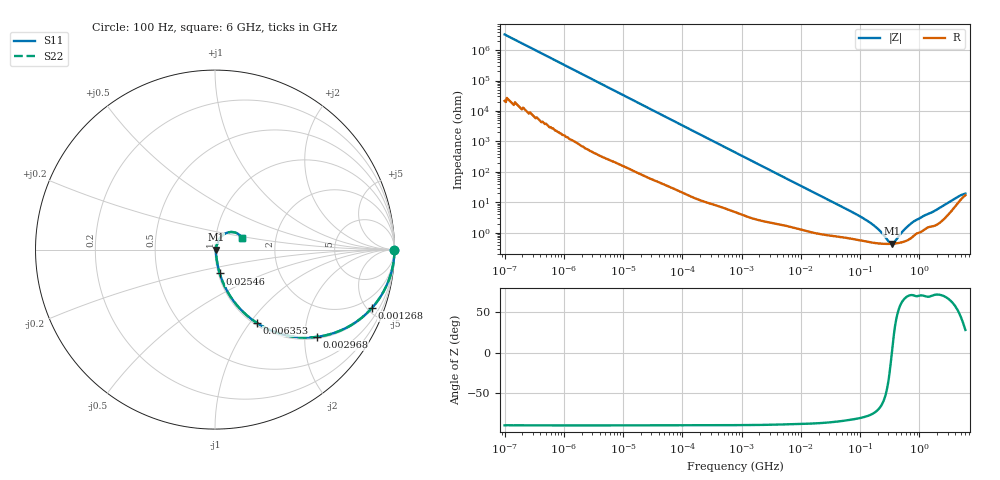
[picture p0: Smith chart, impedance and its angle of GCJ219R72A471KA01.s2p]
!Murata Part Number: GCJ219R72A471KA01
!These Parameters are Measured in Series Mode Connection
!Data Generated on Mar 13, 2026
!  o--ll--o
!Port1  Port2
!  o------o
!Operation Temp=25[degC], DC Bias Voltage=0[V]
!Freq. Start=100[Hz] Stop=6[GHz] 401[Steps]
# Hz S RI R 50
!Freq.(Hz) S11(Real) S11(Imag) S21(Real) S21(Imag) S12(Real) S12(Imag) S22(Real) S22(Imag)
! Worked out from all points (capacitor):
!   401 points, 100 Hz to 6 GHz, reference 50 ohm
!   read as one part in series: C = 484 pF near 109 Hz
!   lowest |Z| = 431 mohm at 341.7 MHz (marker M1)
!   series resonance near 344.2 MHz, so ESL is about 440 pH
!   S11 on the Smith chart (normalised r, x): 100 Hz: open; 1.268 MHz: 1.07, -5.37; 2.968 MHz: 1.04, -2.30; 6.353 MHz: 1.03, -1.09; 25.46 MHz: 1.02, -0.28; 6 GHz: 1.34, +0.18
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100  1 -3.05e-05  2e-07 3.05e-05  2e-07 3.05e-05  1 -3.05e-05
335  1 -0.000101  6e-07 0.000101  6e-07 0.000101  1 -0.000101
2008  1 -0.000604  2.9e-06 0.000604  2.9e-06 0.000604  1 -0.000604
40335  0.9998 -0.012  0.00021 0.012  0.00021 0.012  0.9998 -0.012
241822  0.9944 -0.0713  0.00563 0.0713  0.00563 0.0713  0.9944 -0.0713
774597  0.9484 -0.2159  0.0516 0.2159  0.0516 0.2159  0.9484 -0.2159
1267578  0.8751 -0.3245  0.1249 0.3245  0.1249 0.3245  0.8751 -0.3245
1896632  0.7605 -0.4196  0.2395 0.4196  0.2395 0.4196  0.7605 -0.4196
2967816  0.569 -0.4859  0.431 0.4859  0.431 0.4859  0.569 -0.4859
6353432  0.2341 -0.4091  0.7659 0.4091  0.7659 0.4091  0.2341 -0.4091
1.555665e7  0.0565 -0.2095  0.9435 0.2095  0.9435 0.2095  0.0565 -0.2095
2.545746e7  0.0265 -0.1328  0.9735 0.1328  0.9735 0.1328  0.0265 -0.1328
1.395531e8  0.00541 -0.0223  0.9946 0.0223  0.9946 0.0223  0.00541 -0.0223
2.088084e8  0.00452 -0.0114  0.9955 0.0114  0.9955 0.0114  0.00452 -0.0114
3.124326e8  0.00426 -0.00215  0.9957 0.00215  0.9957 0.00215  0.00426 -0.00215
3.417016e8  0.00429 -0.00016  0.9957 0.00016  0.9957 0.00016  0.00429 -0.00016
3.737127e8  0.00435 0.00184  0.9957 -0.00184  0.9957 -0.00184  0.00435 0.00184
5.59173e8  0.00521 0.0114  0.9948 -0.0114  0.9948 -0.0114  0.00521 0.0114
8.000355e8  0.00816 0.0215  0.9918 -0.0215  0.9918 -0.0215  0.00816 0.0215
2.679998e9  0.034 0.0722  0.966 -0.0722  0.966 -0.0722  0.034 0.0722
4.586474e9  0.1007 0.0975  0.8993 -0.0975  0.8993 -0.0975  0.1007 0.0975
6e9  0.15 0.065  0.85 -0.065  0.85 -0.065  0.15 0.065
